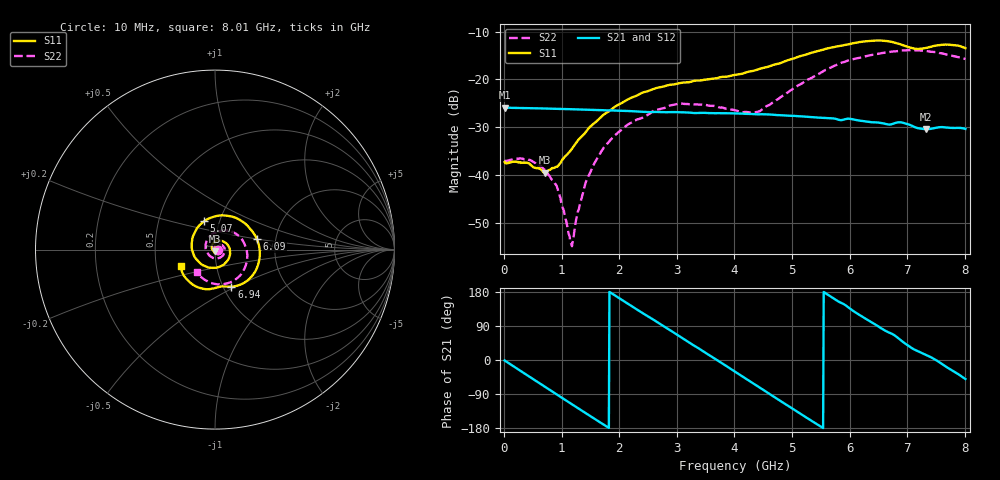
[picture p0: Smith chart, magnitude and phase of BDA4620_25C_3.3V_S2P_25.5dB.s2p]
!Agilent Technologies,E5071B,MY42404982,A.09.10
!Date: Wed May 06 08:54:21 2026
!Data & Calibration Information:
!Freq	S11:SOLT2(ON)	S21:SOLT2(ON)	S12:SOLT2(ON)	S22:SOLT2(ON)
# Hz S RI R 50
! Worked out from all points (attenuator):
!   801 points, 10 MHz to 8.01 GHz, reference 50 ohm
!   highest |S21| = -25.88 dB at 10 MHz (marker M1); lowest = -30.4 dB at 7.33 GHz (marker M2)
!   lowest |S11| = -39.5 dB at 710 MHz (marker M3), VSWR 1.02, Z = 49.8 - j1.04 ohm
!   |S11| at or under -10 dB: start of sweep to end of sweep
!   |S22| runs from -54.9 to -13.9 dB; largest |S21 - S12| = 0.00022
!   S11 on the Smith chart (normalised r, x): 10 MHz: 1.03, -0.00; 5.07 GHz: 0.84, +0.27; 6.09 GHz: 1.59, +0.20; 6.94 GHz: 1.09, -0.48; 8.01 GHz: 0.67, -0.13
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1e7  0.0137 -0.000863  0.0508 -0.00104  0.0509 -0.00109  0.014 -0.000489
4.4e8  0.00847 -0.0101  0.036 -0.0348  0.036 -0.0348  0.0135 -0.00512
7.1e8  -0.00187 -0.0104  0.0164 -0.0469  0.0164 -0.0469  0.00867 -0.00714
9.3e8  -0.011 -0.00553  -0.00201 -0.0492  -0.00206 -0.0493  0.00354 -0.00629
1.16e9  -0.0172 0.00604  -0.0206 -0.0442  -0.0207 -0.0443  -0.00151 -0.00122
1.2e9  -0.0177 0.0085  -0.0235 -0.0426  -0.0236 -0.0426  -0.00209 -3.14e-06
1.35e9  -0.0177 0.0183  -0.0334 -0.0351  -0.0334 -0.0351  -0.0036 0.00455
1.53e9  -0.0127 0.0309  -0.042 -0.0232  -0.0421 -0.0233  -0.00347 0.0112
1.77e9  0.00202 0.0444  -0.0473 -0.00461  -0.0474 -0.00459  0.000629 0.0205
2.15e9  0.0389 0.048  -0.0399 0.0244  -0.0399 0.0245  0.0169 0.0293
2.68e9  0.082 0.00439  -0.00635 0.0451  -0.00628 0.0452  0.0444 0.0197
3.08e9  0.075 -0.0535  0.0231 0.039  0.0233 0.0389  0.0553 -0.00721
4.01e9  -0.0765 -0.0811  0.0379 -0.0226  0.0379 -0.0226  -0.0104 -0.0465
4.42e9  -0.1278 -8.99e-05  0.0144 -0.0407  0.0143 -0.0408  -0.0445 -0.0128
5.07e9  -0.0608 0.1575  -0.0289 -0.0296  -0.029 -0.0297  -0.0228 0.0806
5.35e9  0.022 0.1895  -0.0382 -0.0127  -0.0383 -0.0128  0.023 0.1018
6.09e9  0.2332 0.0589  -0.0226 0.0303  -0.0227 0.0304  0.1583 0.044
6.68e9  0.1821 -0.1715  0.01 0.0322  0.01 0.0323  0.1703 -0.0904
6.94e9  0.0917 -0.2067  0.0243 0.0252  0.0243 0.0253  0.137 -0.1475
7.33e9  0.00346 -0.2133  0.0294 0.00676  0.0294 0.00686  0.0451 -0.1928
7.66e9  -0.1092 -0.2038  0.0302 -0.00891  0.0303 -0.00891  -0.0353 -0.1804
8.01e9  -0.1917 -0.0905  0.0195 -0.0233  0.0196 -0.0233  -0.102 -0.1274
